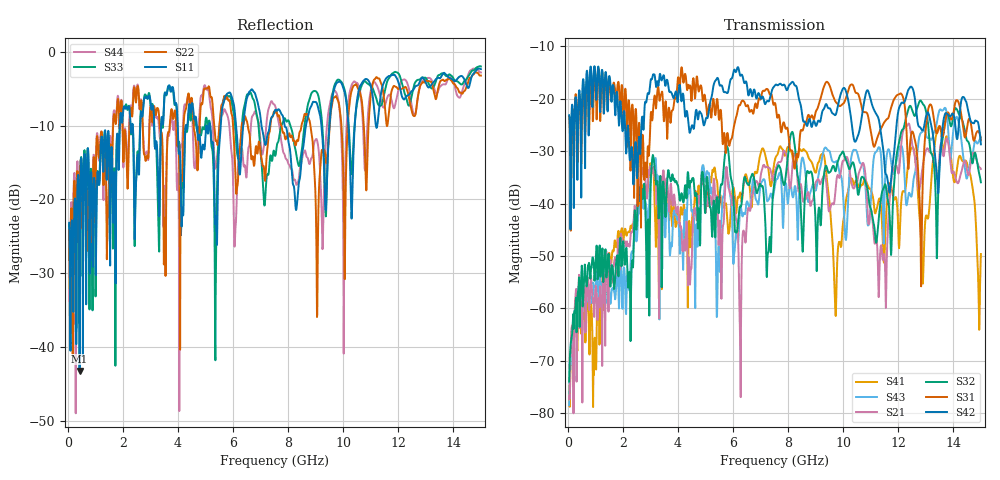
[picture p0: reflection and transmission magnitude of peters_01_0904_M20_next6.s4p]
# MHZ S RI R 50.00
! FREQ  S11  S12  S13  S14
!  S21  S22  S23  S24
!  S31  S32  S33  S34
!  S41  S42  S43  S44
!  REAL  IMAG  REAL  IMAG  REAL  IMAG  REAL  IMAG
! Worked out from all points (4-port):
!   1496 points, 50 MHz to 15 GHz, reference 50 ohm
!   strongest paths, dB at 50 MHz, 3.79 GHz, 7.53 GHz, 11.27 GHz, 15 GHz:
!     S42: -23.1, -19.1, -17.4, -23.5, -28.7
!     S31: -23.4, -22.2, -20.8, -27.0, -27.9
!     S32: -74.0, -34.5, -34.9, -44.1, -35.9
!     S21: -77.4, -39.6, -33.7, -53.9, -33.4
!     S43: -78.5, -47.5, -36.2, -29.4, -27.4
!     S41: -74.7, -44.3, -31.5, -39.8, -49.6
!   lowest |S11| = -43.2 dB at 430 MHz (marker M1), VSWR 1.01, Z = 50.3 + j0.64 ohm
!   |S11| at or under -10 dB: start of sweep to 1.891 GHz; 5.173 GHz to 5.554 GHz (381.1 MHz wide, 7.1 % of centre); 7.874 GHz to 8.649 GHz (775.4 MHz wide, 9.39 % of centre)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
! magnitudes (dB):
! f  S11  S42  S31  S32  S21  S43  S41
! 50 MHz  -23.2  -23.1  -23.4  -74.0  -77.4  -78.5  -74.7
! 430 MHz  -43.2  -18.6  -19.4  -63.5  -63.6  -63.0  -59.5
! 3.03 GHz  -7.7  -16.2  -22.5  -34.1  -34.2  -33.7  -33.0
! 6.26 GHz  -16.4  -15.6  -21.2  -40.5  -66.5  -41.0  -37.9
! 12.89 GHz  -3.5  -26.0  -36.0  -20.9  -32.7  -26.2  -55.3
! 13.48 GHz  -3.6  -35.5  -25.4  -34.1  -31.9  -22.4  -25.2
! 15 GHz  -2.4  -28.7  -27.9  -35.9  -33.4  -27.4  -49.6
